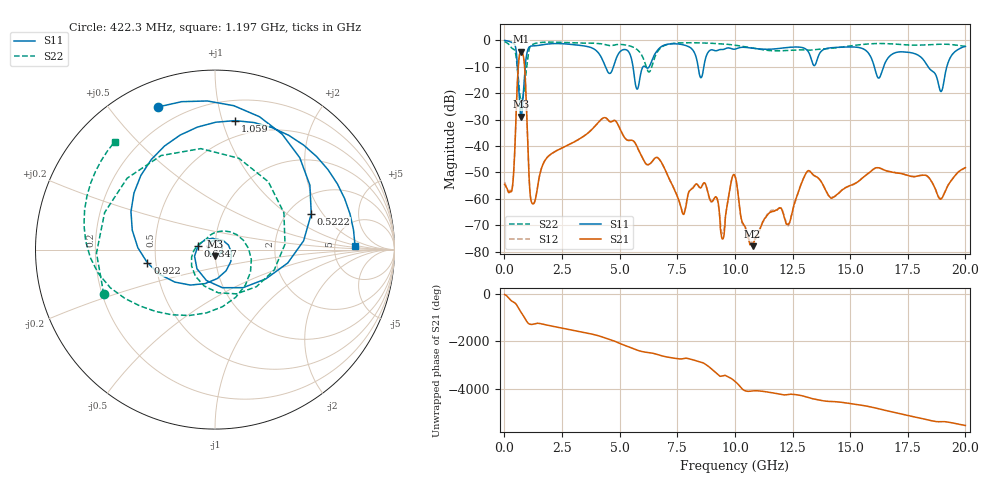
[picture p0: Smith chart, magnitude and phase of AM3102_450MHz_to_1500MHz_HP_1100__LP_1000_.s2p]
!Agilent Technologies,E8364B,MY43040894,A.07.50.67
!Agilent E8364B: A.07.50.67
!Date: Thursday, January 11, 2018 06:34:04
!Correction: S11(Full 2 Port(1,2))
!S21(Full 2 Port(1,2))
!S12(Full 2 Port(1,2))
!S22(Full 2 Port(1,2))
!S2P File: Measurements: S11, S21, S12, S22:
# Hz S  dB  R 50
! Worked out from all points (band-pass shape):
!   1601 points, 10 MHz to 20 GHz, reference 50 ohm
!   highest |S21| = -4.32 dB at 722.1 MHz (marker M1); lowest = -77.9 dB at 10.77 GHz (marker M2)
!   |S21| within 3 dB of the highest: 629.8 MHz to 848.2 MHz (218.4 MHz wide, 29.6 % of centre)
!   lowest |S11| = -28.9 dB at 722.1 MHz (marker M3), VSWR 1.07, Z = 49.7 - j3.56 ohm
!   |S11| at or under -10 dB: 5.58 GHz to 6.018 GHz (437.7 MHz wide, 7.55 % of centre); 16.05 GHz to 16.45 GHz (401.2 MHz wide, 2.47 % of centre); 18.38 GHz to 19.2 GHz (816.4 MHz wide, 4.35 % of centre)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
!   |S22| runs from -22.6 to -0.5 dB; largest |S21 - S12| = 0.0014
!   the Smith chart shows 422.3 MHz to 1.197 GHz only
!   S11 on the Smith chart (normalised r, x): 422.3 MHz: 0.11, +0.67; 522.2 MHz: 2.64, +1.56; 634.7 MHz: 0.83, +0.04; 922 MHz: 0.45, -0.08; 1.059 GHz: 0.36, +1.10; 1.197 GHz: 8.02, +0.85
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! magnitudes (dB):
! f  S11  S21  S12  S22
! 10 MHz  -0.1  -54.5  -53.6  -0.5
! 422.3 MHz  -1.4  -47.0  -47.1  -3.5
! 522.2 MHz  -4.8  -24.5  -24.5  -7.2
! 634.7 MHz  -20.2  -6.9  -6.9  -17.3
! 722.1 MHz  -28.9  -4.3  -4.3  -22.6
! 922 MHz  -8.3  -17.3  -17.3  -13.6
! 1.059 GHz  -2.8  -49.4  -49.4  -4.1
! 1.197 GHz  -2.2  -61.6  -61.4  -1.7
! 3.346 GHz  -2.0  -36.9  -36.8  -1.1
! 5.32 GHz  -3.8  -37.7  -37.7  -1.9
! 5.757 GHz  -18.5  -40.3  -40.3  -3.5
! 6.682 GHz  -3.4  -44.7  -44.6  -3.8
! 7.744 GHz  -1.7  -65.8  -65.4  -1.0
! 8.706 GHz  -7.6  -54.1  -54.1  -1.0
! 9.468 GHz  -3.5  -75.2  -73.1  -1.4
! 10.01 GHz  -3.4  -51.4  -51.3  -1.9
! 10.77 GHz  -3.0  -77.9  -76.8  -3.0
! 13.34 GHz  -8.0  -50.4  -50.4  -3.7
! 14.22 GHz  -2.8  -59.7  -59.3  -3.0
! 16.68 GHz  -6.4  -49.6  -49.6  -1.3
! 18.94 GHz  -19.4  -60.1  -59.8  -1.5
! 20 GHz  -2.3  -48.2  -48.3  -2.3
